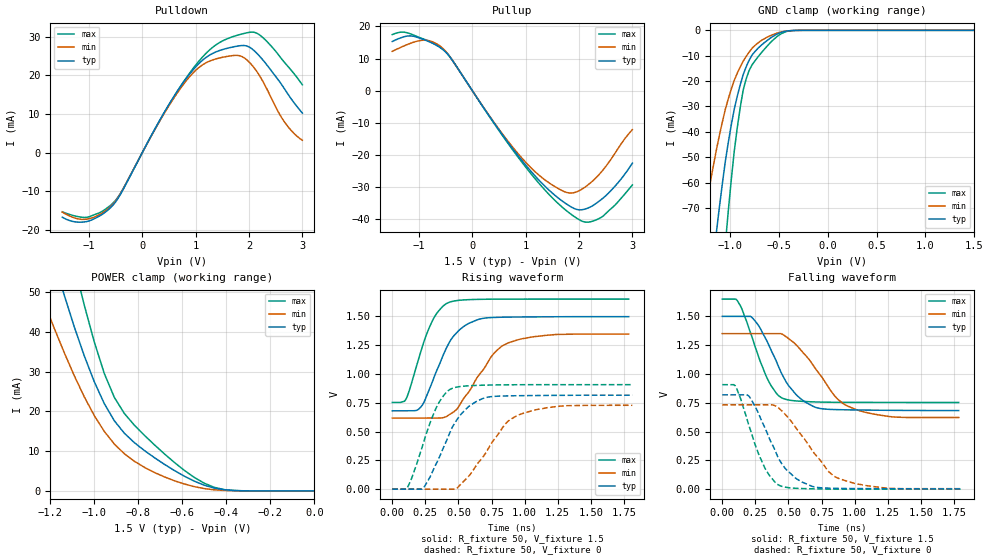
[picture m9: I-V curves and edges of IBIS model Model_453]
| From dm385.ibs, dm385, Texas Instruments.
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| Model based on original model for BCSHTLTCSCDDVPBFZ_SSDHV
|   Sub model SR10_9MA_PADN_10PER_1P5
[model]   Model_453
|[Description]  [1.5V-3-STATE-NOTERM-SLOW:9MA, IND, 10%]
|   Slow slew rate (SR[1:0] = "01"), 0.88 * RExt = 1.125 * Iout
|   (I[2:0] = "100"), 9mA nominal with Rext = 50R,ODT off (ODT[1:0]
|   = "00") CMOS mode,Industrial temperature range (-40C to 125C,
|   25C nominal),10% power supply tolerance
|[Input Load]   NOTERM
|[Output Drive] SLOW:9MA
|Voltage   1.5V
|Mode   3-STATE
Model_type   3-state
Polarity   Non-Inverting
Enable   Active-Low
Cref =  15pF
Rref =  100.0000M
Vref =  0V
Vmeas =  0.75
C_comp   1.865048p   1.676829p   1.989968p
[Temperature Range]   25   125   -40
[Voltage Range]   1.5   1.35   1.65
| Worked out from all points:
|   slope of the pulldown table from 0 to 0.225 V, typ, clamps not added: 38.4 ohm
|   slope of the pullup table from 0 to 0.225 V, typ, clamps not added: 40.1 ohm
|   GND clamp passes 1 mA (typ) near -0.49 V on its own axis
|   POWER clamp passes 1 mA (typ) near -0.47 V on its own axis
|   rising waveform, R_fixture 50, V_fixture 1.5: 20-80 % time 196ps typ, 261ps min, 159ps max; typ from 0.68 V to 1.5 V
|   rising waveform, R_fixture 50, V_fixture 0: 20-80 % time 213ps typ, 268ps min, 167ps max; typ from 0 V to 0.816 V
|   falling waveform, R_fixture 50, V_fixture 1.5: 20-80 % time 225ps typ, 290ps min, 174ps max; typ from 1.5 V to 0.682 V
|   falling waveform, R_fixture 50, V_fixture 0: 20-80 % time 213ps typ, 284ps min, 168ps max; typ from 0.818 V to 0.003 V
[POWER_clamp]
-1.5V     126mA      88.79mA    168.7mA
-1.242V   69.8mA     49.45mA    94.34mA
-1.136V   49.16mA    34.72mA    67.51mA
-1.061V   36.35mA    25.4mA     50.03mA
-1.045V   33.92mA    23.63mA    46.66mA
-954.5mV  21.93mA    14.95mA    29.5mA
-909.1mV  17.64mA    11.79mA    23.52mA
-863.6mV  14.51mA    9.351mA    19.47mA
-772.7mV  10.16mA    5.94mA     13.99mA
-590.9mV  3.705mA    1.741mA    5.166mA
-454.5mV  710.5uA    279.1uA    892.1uA
0V        1.424nA    14.34nA    3.127nA
[Pulldown]
-1.5V     -16.73mA   -15.43mA   -15.34mA
-1V       -17.72mA   -17.14mA   -16.64mA
-727.3mV  -15.78mA   -15.46mA   -14.99mA
-500mV    -12.78mA   -12.54mA   -12.34mA
272.7mV   7.051mA    6.89mA     6.983mA
681.8mV   16.43mA    15.99mA    16.46mA
1.045V    22.87mA    21.88mA    23.45mA
1.364V    26mA       24.22mA    27.76mA
1.818V    27.68mA    25.13mA    30.56mA
2.136V    25.9mA     21.22mA    31.01mA
2.636V    17.13mA    8.517mA    23.85mA
3V        10.24mA    3.203mA    17.58mA
[Pullup]
-1.5V     15.3mA     12.24mA    17.45mA
-1.182V   17.04mA    14.59mA    17.8mA
-954.5mV  16.15mA    15.65mA    16.31mA
-590.9mV  13.28mA    13.71mA    13.34mA
-409.1mV  10.24mA    10.29mA    10.33mA
909.1mV   -21.29mA   -20.6mA    -21.82mA
1.318V    -29.04mA   -27.22mA   -30.13mA
1.773V    -35.35mA   -31.7mA    -37.46mA
2.045V    -37.08mA   -30.75mA   -40.54mA
2.318V    -35.11mA   -27.11mA   -40.23mA
2.682V    -29.59mA   -19.28mA   -35.49mA
3V        -22.57mA   -12.13mA   -29.35mA
[GND_clamp]
-1.5V     -219.3mA   -131.6mA   -364.3mA
-1.288V   -134.4mA   -79.74mA   -225.6mA
-1.258V   -122.9mA   -72.77mA   -206.3mA
-1.136V   -79.27mA   -46.88mA   -132.4mA
-1.045V   -51.5mA    -31.06mA   -84.11mA
-1.015V   -44.02mA   -26.9mA    -70.91mA
-954.5mV  -31.01mA   -19.7mA    -47.55mA
-863.6mV  -17.48mA   -12.16mA   -23.55mA
-803mV    -11.81mA   -8.597mA   -15.85mA
-681.8mV  -5.986mA   -4.096mA   -9.026mA
-378.8mV  -126.2uA   -131.8uA   -179.7uA
1.5V      1.424nA    207.1nA    1.498nA
[Ramp]
dV/dt_f  0.4938488/0.2273583n 0.44129726/0.29322266n 0.54002912/0.17416198n
dV/dt_r 0.49361865/0.21530402n 0.44147722/0.27016875n  0.5459917/0.16779954n
R_load = 50
[Rising Waveform]
R_fixture = 50
V_fixture = 1.5
V_fixture_min = 1.35
V_fixture_max = 1.65
0s        680.2mV    616.8mV    752.8mV
103.9ps   680.2mV    616.8mV    781.5mV
216.8ps   714.8mV    616.8mV    1.198V
323.8ps   996.1mV    617.3mV    1.505V
433.4ps   1.279V     648.4mV    1.623V
631.5ps   1.465V     951mV      1.647V
761.6ps   1.49V      1.17V      1.649V
877.4ps   1.493V     1.27V      1.65V
1.241ns   1.496V     1.343V     1.65V
1.787ns   1.497V     1.346V     1.65V
[Rising Waveform]
R_fixture = 50
V_fixture = 0
V_fixture_min = 0
V_fixture_max = 0
0s        0V         0V         0V
116.3ps   0V         0V         18.01mV
232.6ps   7.422mV    0V         390.9mV
342.2ps   244.1mV    0V         729.8mV
451ps     531.7mV    0V         874.2mV
643.7ps   765.7mV    220.2mV    900.9mV
852.9ps   809.1mV    564.9mV    905.7mV
967.9ps   811.4mV    650.6mV    906.5mV
1.308ns   814.5mV    724.2mV    906.8mV
1.814ns   815.5mV    728.1mV    907.1mV
[Falling Waveform]
R_fixture = 50
V_fixture = 1.5
V_fixture_min = 1.35
V_fixture_max = 1.65
0s        1.499V     1.349V     1.649V
113.8ps   1.499V     1.349V     1.635V
222.1ps   1.492V     1.349V     1.328V
339.7ps   1.28V      1.349V     961mV
458.1ps   982.2mV    1.341V     787.6mV
560.4ps   817.3mV    1.249V     765.2mV
668.9ps   728.9mV    1.105V     758.1mV
937.7ps   688.4mV    725.9mV    753mV
1.26ns    684mV      630.2mV    752.2mV
1.787ns   682.2mV    621.8mV    751.8mV
[Falling Waveform]
R_fixture = 50
V_fixture = 0
V_fixture_min = 0
V_fixture_max = 0
0s        818.4mV    731.6mV    906.3mV
98.4ps    818.4mV    731.6mV    896.4mV
205.4ps   801.6mV    731.6mV    537.6mV
324.7ps   525.8mV    731.6mV    176.9mV
433.7ps   249.3mV    695.9mV    31.29mV
603.3ps   61.36mV    460.7mV    5.334mV
799.9ps   8.867mV    156mV      0V
883ps     6.711mV    91.21mV    0V
1.254ns   3.789mV    7.479mV    0V
1.814ns   2.676mV    4.245mV    0V
